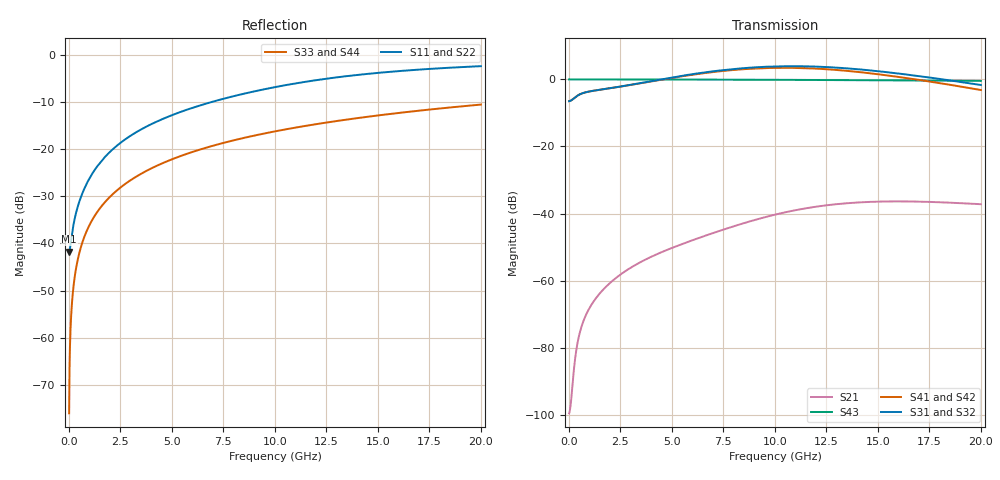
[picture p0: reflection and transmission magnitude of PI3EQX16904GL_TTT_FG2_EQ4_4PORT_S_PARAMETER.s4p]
! NPort=4 DATA=2000 NOISE=0 GROUPDELAY=0 COMPLEX_DATAFORMAT=POLAR
! NumOfBlock=1 NumOfParam=0
! .MODEL Smodel S TSTONEFILE=PI3EQX16904GL_TTT_FG2_EQ4_4PORT_S_PARAMETER.s4p TYPE=S
!  -- The above .MODEL line can be used for the S element in the netlist.
! The s parameter is extracted from the linear redriver, it is not bi-directional; only s(4,1)s(4,2) and s(3,1)s(3,2)
! should be the insertion loss
!Port definition:
!Port1 = input+
!Port2 = input-
!Port3 = output+
!Port4 = output-
# Hz S MA R  50
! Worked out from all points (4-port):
!   2000 points, 10 MHz to 20 GHz, reference 50 ohm
!   strongest paths, dB at 10 MHz, 5.01 GHz, 10.01 GHz, 15.01 GHz, 20 GHz:
!     S31: -6.5, 0.6, 3.9, 2.4, -1.7
!     S32: -6.5, 0.4, 3.6, 2.2, -1.9
!     S41: -6.5, 0.5, 3.5, 1.5, -3.2
!     S42: -6.5, 0.3, 3.2, 1.3, -3.4
!     S43: 0.0, 0.0, -0.1, -0.3, -0.4
!     S21: -99.6, -50.2, -40.3, -36.4, -37.2
!   lowest |S11| = -41.7 dB at 10 MHz (marker M1), VSWR 1.02, Z = 49.2 - j0.0603 ohm
!   |S11| at or under -10 dB: start of sweep to 6.893 GHz
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1e7  0.008182 -175.7  1.05e-05 7.7  0 0.0  0 0.0
     1.05e-05 7.7  0.008182 -175.7  0 0.0  0 0.0
     0.4743 0.4  0.4743 -179.6  0.0001571 -90.0  1 -0.0
     0.4743 -179.6  0.4743 0.4  1 -0.0  0.0001571 -90.0
3.9e8  0.02299 -119.3  0.0001055 117.7  0 0.0  0 0.0
       0.0001055 117.7  0.02299 -119.3  0 0.0  0 0.0
       0.5668 9.5  0.5663 -170.7  0.006126 -90.4  1 -0.4
       0.5667 -171.2  0.5663 8.6  1 -0.4  0.006126 -90.4
1.64e9  0.07788 -102.7  0.000721 106.5  0 0.0  0 0.0
        0.0007209 106.5  0.07788 -102.7  0 0.0  0 0.0
        0.7124 1.1  0.7101 -179.5  0.02575 -91.5  0.9996 -1.5
        0.7115 178.1  0.7091 -2.5  0.9996 -1.5  0.02575 -91.5
6.1e9  0.2801 -105.2  0.004133 87.7  0 0.0  0 0.0
       0.004105 87.8  0.2801 -105.2  0 0.0  0 0.0
       1.211 -40.1  1.175 139.2  0.09535 -95.7  0.9951 -5.5
       1.188 129.1  1.154 -51.6  0.9951 -5.5  0.09535 -95.7
9.96e9  0.4557 -112.8  0.009639 60.5  0 0.0  0 0.0
        0.009551 61.2  0.4552 -112.8  0 0.0  0 0.0
        1.561 -98.9  1.517 81.0  0.1544 -99.2  0.987 -8.9
        1.487 63.8  1.445 -116.3  0.987 -8.9  0.1544 -99.2
1.407e10  0.6185 -123.1  0.01473 16.1  0 0.0  0 0.0
          0.01465 17.2  0.6178 -123.1  0 0.0  0 0.0
          1.414 -166.3  1.379 13.7  0.2154 -102.9  0.9746 -12.4
          1.289 -10.1  1.257 169.9  0.9746 -12.4  0.2154 -102.9
2e10  0.7637 -136.0  0.01381 -35.1  0 0.0  0 0.0
      0.01378 -33.5  0.7634 -135.9  0 0.0  0 0.0
      0.8258 111.2  0.8061 -68.8  0.2986 -108.1  0.9506 -17.4
      0.6953 -100.7  0.6788 79.3  0.9506 -17.4  0.2986 -108.1
